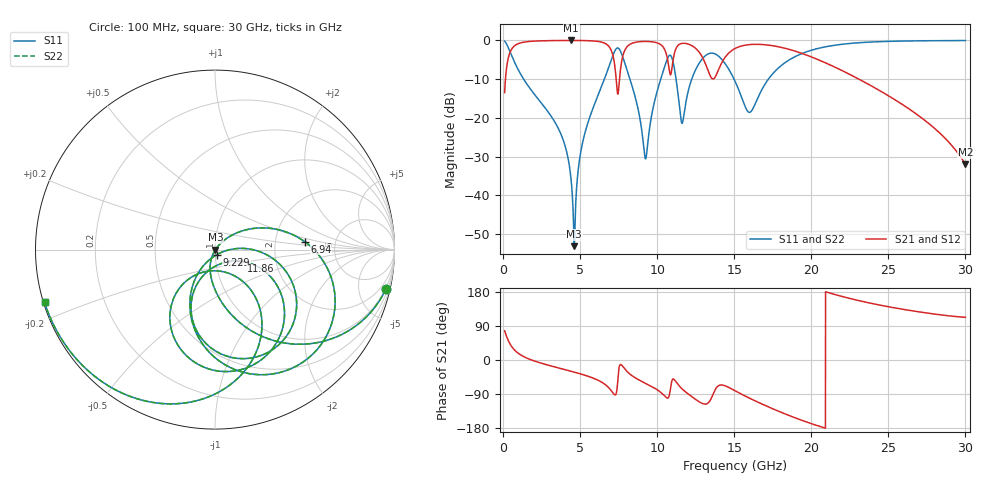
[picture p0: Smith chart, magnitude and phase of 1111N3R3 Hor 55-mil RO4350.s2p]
# GHz S MA R 50
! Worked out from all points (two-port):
!   3201 points, 100 MHz to 30 GHz, reference 50 ohm
!   highest |S21| = -0.02 dB at 4.417 GHz (marker M1); lowest = -31.9 dB at 30 GHz (marker M2)
!   |S21| within 3 dB of the highest: 459.5 MHz to 7.061 GHz (6.602 GHz wide, 176 % of centre); 14.71 GHz to 19.14 GHz (4.432 GHz wide, 26.2 % of centre)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
!   lowest |S11| = -53.1 dB at 4.622 GHz (marker M3), VSWR 1.00, Z = 50.2 - j0.107 ohm
!   |S11| at or under -10 dB: 1.336 GHz to 6.574 GHz (5.238 GHz wide, 132 % of centre); 8.232 GHz to 10.23 GHz (1.998 GHz wide, 21.6 % of centre); 14.99 GHz to 17.22 GHz (2.228 GHz wide, 13.8 % of centre)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
!   |S22| runs from -53.1 to 0.0 dB; largest |S21 - S12| = 0
!   S11 on the Smith chart (normalised r, x): 100 MHz: 0.90, -8.74; 6.94 GHz: 2.97, +0.35; 9.229 GHz: 1.02, -0.06; 11.86 GHz: 1.33, -0.18; 30 GHz: 0.00, -0.15
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0.1  0.9773 -12.9  0.2115 77.1  0.2115 77.1  0.9773 -12.9
1.211906  0.3471 -78.1  0.937 11.8  0.937 11.8  0.3471 -78.1
3.669313  0.06761 -110.5  0.9959 -21.7  0.9959 -21.7  0.06761 -110.5
4.416812  0.01577 -112.5  0.9974 -29.7  0.9974 -29.7  0.01577 -112.5
4.622375  0.00222 -28.8  0.9973 -32.0  0.9973 -32.0  0.00222 -28.8
5.089563  0.04102 48.2  0.9955 -37.5  0.9955 -37.5  0.04102 48.2
6.939625  0.5016 5.1  0.7973 -77.0  0.7973 -77.0  0.5016 5.1
7.294688  0.7559 -28.8  0.3944 -91.8  0.3944 -91.8  0.7559 -28.8
7.603031  0.7358 -71.2  0.3959 -12.2  0.3959 -12.2  0.7358 -71.2
8.079562  0.3941 -109.9  0.8414 -31.6  0.8414 -31.6  0.3941 -109.9
9.228844  0.02983 -68.9  0.9694 -61.2  0.9694 -61.2  0.02983 -68.9
10.06978  0.2472 -2.5  0.9177 -80.5  0.9177 -80.5  0.2472 -2.5
10.90137  0.6291 -75.0  0.3731 -65.2  0.3731 -65.2  0.6291 -75.0
11.56478  0.08999 -85.7  0.9104 -74.2  0.9104 -74.2  0.08999 -85.7
11.86378  0.159 -24.2  0.9113 -84.9  0.9113 -84.9  0.159 -24.2
12.8075  0.5367 -43.9  0.6675 -112.3  0.6675 -112.3  0.5367 -43.9
13.58303  0.684 -82.9  0.319 -94.5  0.319 -94.5  0.684 -82.9
15.05  0.2978 -132.5  0.7854 -81.1  0.7854 -81.1  0.2978 -132.5
16.03109  0.1185 -86.1  0.8837 -101.6  0.8837 -101.6  0.1185 -86.1
20.03956  0.7494 -82.5  0.6084 -168.5  0.6084 -168.5  0.7494 -82.5
25.01978  0.9709 -132.0  0.1924 140.4  0.1924 140.4  0.9709 -132.0
30  0.9943 -162.8  0.02528 112.7  0.02528 112.7  0.9943 -162.8
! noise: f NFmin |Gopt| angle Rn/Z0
0.1  0.001363  0.8748  3.365  0.002347
3.417  0.009524  0.4703  25.3  0.002916
6.743  0.07058  0.8299  45.45  0.07448
10.06  0.0958  0.8202  66.11  0.07877
13.39  0.5561  0.957  85.45  1.577
16.7  0.1649  0.8342  103.1  0.08234
20.03  0.1652  0.8105  118.3  0.04918
23.35  0.2304  0.8492  132.9  0.05373
26.67  0.4284  0.9146  148  0.08621
30  1.625  0.9772  163.4  0.3463
